| IBIS file stm32l4r5_s5_r7_s7_lqfp144.ibs
[IBIS ver]   4.2
[File name]   stm32l4r5_s5_r7_s7_lqfp144.ibs
[File Rev]   1.0
[Date]   01-6-2017
[Source]   Data Created at STMicroelectronics
[Notes]   File originated from ELDO simulations.
[Disclaimer]  This information is for modeling purpose only and is
   not guaranted.
   The information is subject to change without notice.
[Copyright]   Copyright 2017 STMicroelectronics Inc.
|   Component stm32l4r5_s5_r7_s7_lqfp144
[Component] stm32l4r5_s5_r7_s7_lqfp144
[Manufacturer] STMicroelectronics
[Package]
| variable   typ   min   max
R_pkg   0.0   0.0   0.0
L_pkg   0.0H   0.0H   0.0H
C_pkg   0.0F   0.0F   0.0F
[Pin]  signal_name   model_name   R_pin   L_pin   C_pin
1 PE2 io8prog2m25m50m120m_sudq_ft 187.6E-3 9.4E-9 267.9E-15
2 PE3 io8prog2m25m50m120m_sudq_ft 182.4E-3 9.1E-9 243.8E-15
3 PE4 io8prog2m25m50m120m_sudq_ft 177.6E-3 8.7E-9 221.3E-15
4 PE5 io8prog2m25m50m120m_sudq_ft 173.1E-3 8.4E-9 200.2E-15
5 PE6 io8prog2m25m50m120m_sudq_ft 168.9E-3 8.1E-9 180.5E-15
6 VBAT power 165.0E-3 7.8E-9 162.3E-15
7 PC13 io8prog2m25m50m120m_sudq_ft 161.5E-3 7.6E-9 145.6E-15
8 PC14-OSC32_IN io8prog2m25m50m120m_sudq_ft 158.2E-3 7.4E-9 130.3E-15
9 PC15-OSC32_OUT io8prog2m25m50m120m_sudq_ft 155.2E-3 7.2E-9 116.4E-15
10 PF0 io8prog2m25m50m120m_sudq_i2c_ft 152.6E-3 7.0E-9 104.1E-15
11 PF1 io8prog2m25m50m120m_sudq_i2c_ft 150.3E-3 6.8E-9 93.2E-15
12 PF2 io8prog2m25m50m120m_sudq_ft 148.2E-3 6.7E-9 83.7E-15
13 PF3 io8prog2m25m50m120m_sudq_ft 146.5E-3 6.5E-9 75.7E-15
14 PF4 io8prog2m25m50m120m_sudq_ft 145.1E-3 6.4E-9 69.1E-15
15 PF5 io8prog2m25m50m120m_sudq_ft 144.1E-3 6.4E-9 64.0E-15
16 VSS gnd 143.3E-3 6.3E-9 60.4E-15
17 VDD power 142.8E-3 6.3E-9 58.2E-15
18 PF6 io8prog2m25m50m120m_sudq_ft 142.7E-3 6.3E-9 57.5E-15
19 PF7 io8prog2m25m50m120m_sudq_ft 142.7E-3 6.3E-9 57.5E-15
20 PF8 io8prog2m25m50m120m_sudq_ft 142.8E-3 6.3E-9 58.2E-15
21 PF9 io8prog2m25m50m120m_sudq_ft 143.3E-3 6.3E-9 60.4E-15
22 PF10 io8prog2m25m50m120m_sudq_ft 144.1E-3 6.4E-9 64.0E-15
23 PH0-OSC_IN io8prog2m25m50m120m_sudq_ft 145.1E-3 6.4E-9 69.1E-15
24 PH1-OSC_OUT io8prog2m25m50m120m_sudq_ft 146.5E-3 6.5E-9 75.7E-15
25 NRST ioreset_ft_v33 148.2E-3 6.7E-9 83.7E-15
26 PC0 io8prog2m25m50m120m_sudq_i2c_ft 150.3E-3 6.8E-9 93.2E-15
27 PC1 io8prog2m25m50m120m_sudq_i2c_ft 152.6E-3 7.0E-9 104.1E-15
28 PC2 io8prog2m25m50m120m_sudq_ft 155.2E-3 7.2E-9 116.4E-15
29 PC3 io8prog2m25m50m120m_sudq_ft 158.2E-3 7.4E-9 130.3E-15
30 VSSA gnd 161.5E-3 7.6E-9 145.6E-15
31 VREF- gnd 165.0E-3 7.8E-9 162.3E-15
32 VREF+ power 168.9E-3 8.1E-9 180.5E-15
33 VDDA power 173.1E-3 8.4E-9 200.2E-15
34 PA0 io8prog2m25m50m120m_sudq_ft 177.6E-3 8.7E-9 221.3E-15
35 PA1 io8prog2m25m50m120m_sudq_ft 182.4E-3 9.1E-9 243.8E-15
36 PA2 io8prog2m25m50m120m_sudq_ft 187.6E-3 9.4E-9 267.9E-15
37 PA3 io8prog2m25m50m120m_sudq_ft 187.6E-3 9.4E-9 267.9E-15
38 VSS gnd 182.4E-3 9.1E-9 243.8E-15
39 VDD power 177.6E-3 8.7E-9 221.3E-15
40 PA4 io8prog2m25m50m120m_sudq_ft 173.1E-3 8.4E-9 200.2E-15
41 PA5 io8prog2m25m50m120m_sudq_ft 168.9E-3 8.1E-9 180.5E-15
42 PA6 io8prog2m25m50m120m_sudq_ft 165.0E-3 7.8E-9 162.3E-15
43 PA7 io8prog2m25m50m120m_sudq_i2c_ft 161.5E-3 7.6E-9 145.6E-15
44 PC4 io8prog2m25m50m120m_sudq_ft 158.2E-3 7.4E-9 130.3E-15
45 PC5 io8prog2m25m50m120m_sudq_ft 155.2E-3 7.2E-9 116.4E-15
46 PB0 io8prog2m25m50m120m_sudq_ft 152.6E-3 7.0E-9 104.1E-15
47 PB1 io8prog2m25m50m120m_sudq_ft 150.3E-3 6.8E-9 93.2E-15
48 PB2 io8prog2m25m50m120m_sudq_ft 148.2E-3 6.7E-9 83.7E-15
49 PF11 io8prog2m25m50m120m_sudq_ft 146.5E-3 6.5E-9 75.7E-15
50 PF12 io8prog2m25m50m120m_sudq_ft 145.1E-3 6.4E-9 69.1E-15
51 VSS gnd 144.1E-3 6.4E-9 64.0E-15
52 VDD power 143.3E-3 6.3E-9 60.4E-15
53 PF13 io8prog2m25m50m120m_sudq_ft 142.8E-3 6.3E-9 58.2E-15
54 PF14 io8prog2m25m50m120m_sudq_i2c_ft 142.7E-3 6.3E-9 57.5E-15
55 PF15 io8prog2m25m50m120m_sudq_i2c_ft 142.7E-3 6.3E-9 57.5E-15
56 PG0 io8prog2m25m50m120m_sudq_ft 142.8E-3 6.3E-9 58.2E-15
57 PG1 io8prog2m25m50m120m_sudq_ft 143.3E-3 6.3E-9 60.4E-15
58 PE7 io8prog2m25m50m120m_sudq_ft 144.1E-3 6.4E-9 64.0E-15
59 PE8 io8prog2m25m50m120m_sudq_ft 145.1E-3 6.4E-9 69.1E-15
60 PE9 io8prog2m25m50m120m_sudq_ft 146.5E-3 6.5E-9 75.7E-15
61 VSS gnd 148.2E-3 6.7E-9 83.7E-15
62 VDD power 150.3E-3 6.8E-9 93.2E-15
63 PE10 io8prog2m25m50m120m_sudq_ft 152.6E-3 7.0E-9 104.1E-15
64 PE11 io8prog2m25m50m120m_sudq_ft 155.2E-3 7.2E-9 116.4E-15
65 PE12 io8prog2m25m50m120m_sudq_ft 158.2E-3 7.4E-9 130.3E-15
66 PE13 io8prog2m25m50m120m_sudq_ft 161.5E-3 7.6E-9 145.6E-15
67 PE14 io8prog2m25m50m120m_sudq_ft 165.0E-3 7.8E-9 162.3E-15
68 PE15 io8prog2m25m50m120m_sudq_ft 168.9E-3 8.1E-9 180.5E-15
69 PB10 io8prog2m25m50m120m_sudq_i2c_ft 173.1E-3 8.4E-9 200.2E-15
70 PB11 io8prog2m25m50m120m_sudq_i2c_ft 177.6E-3 8.7E-9 221.3E-15
71 VSS gnd 182.4E-3 9.1E-9 243.8E-15
72 VDD power 187.6E-3 9.4E-9 267.9E-15
73 PB12 io8prog2m25m50m120m_sudq_ft 187.6E-3 9.4E-9 267.9E-15
74 PB13 io8prog2m25m50m120m_sudq_i2c_ft 182.4E-3 9.1E-9 243.8E-15
75 PB14 io8prog2m25m50m120m_sudq_i2c_ft 177.6E-3 8.7E-9 221.3E-15
76 PB15 io8prog2m25m50m120m_sudq_ft 173.1E-3 8.4E-9 200.2E-15
77 PD8 io8prog2m25m50m120m_sudq_ft 168.9E-3 8.1E-9 180.5E-15
78 PD9 io8prog2m25m50m120m_sudq_ft 165.0E-3 7.8E-9 162.3E-15
79 PD10 io8prog2m25m50m120m_sudq_ft 161.5E-3 7.6E-9 145.6E-15
80 PD11 io8prog2m25m50m120m_sudq_ft 158.2E-3 7.4E-9 130.3E-15
81 PD12 io8prog2m25m50m120m_sudq_ft 155.2E-3 7.2E-9 116.4E-15
82 PD13 io8prog2m25m50m120m_sudq_ft 152.6E-3 7.0E-9 104.1E-15
83 VSS gnd 150.3E-3 6.8E-9 93.2E-15
84 VDD power 148.2E-3 6.7E-9 83.7E-15
85 PD14 io8prog2m25m50m120m_sudq_ft 146.5E-3 6.5E-9 75.7E-15
86 PD15 io8prog2m25m50m120m_sudq_ft 145.1E-3 6.4E-9 69.1E-15
87 PG2 io8prog2m25m50m120m_sudq_ft 144.1E-3 6.4E-9 64.0E-15
88 PG3 io8prog2m25m50m120m_sudq_ft 143.3E-3 6.3E-9 60.4E-15
89 PG4 io8prog2m25m50m120m_sudq_ft 142.8E-3 6.3E-9 58.2E-15
90 PG5 io8prog2m25m50m120m_sudq_ft 142.7E-3 6.3E-9 57.5E-15
91 PG6 io8prog2m25m50m120m_sudq_ft 142.7E-3 6.3E-9 57.5E-15
92 PG7 io8prog2m25m50m120m_sudq_i2c_ft 142.8E-3 6.3E-9 58.2E-15
93 PG8 io8prog2m25m50m120m_sudq_i2c_ft 143.3E-3 6.3E-9 60.4E-15
94 VSS gnd 144.1E-3 6.4E-9 64.0E-15
95 VDDIO2 power 145.1E-3 6.4E-9 69.1E-15
96 PC6 io8prog2m25m50m120m_sudq_ft 146.5E-3 6.5E-9 75.7E-15
97 PC7 io8prog2m25m50m120m_sudq_ft 148.2E-3 6.7E-9 83.7E-15
98 PC8 io8prog2m25m50m120m_sudq_ft 150.3E-3 6.8E-9 93.2E-15
99 PC9 io8prog2m25m50m120m_sudq_ft 152.6E-3 7.0E-9 104.1E-15
100 PA8 io8prog2m25m50m120m_sudq_ft 155.2E-3 7.2E-9 116.4E-15
101 PA9 power 158.2E-3 7.4E-9 130.3E-15
102 PA10 io8usb_id_otg20_lcd4_ft_ms 161.5E-3 7.6E-9 145.6E-15
103 PA11 io8usblsfs_otg2 165.0E-3 7.8E-9 162.3E-15
104 PA12 io8usblsfs_otg2 168.9E-3 8.1E-9 180.5E-15
105 PA13 io8prog2m25m50m120m_sudq_ft 173.1E-3 8.4E-9 200.2E-15
106 VDDUSB power 177.6E-3 8.7E-9 221.3E-15
107 VSS gnd 182.4E-3 9.1E-9 243.8E-15
108 VDD power 187.6E-3 9.4E-9 267.9E-15
109 PA14 io8prog2m25m50m120m_sudq_ft 187.6E-3 9.4E-9 267.9E-15
110 PA15 io8prog2m25m50m120m_sudq_ft 182.4E-3 9.1E-9 243.8E-15
111 PC10 io8prog2m25m50m120m_sudq_ft 177.6E-3 8.7E-9 221.3E-15
112 PC11 io8prog2m25m50m120m_sudq_ft 173.1E-3 8.4E-9 200.2E-15
113 PC12 io8prog2m25m50m120m_sudq_ft 168.9E-3 8.1E-9 180.5E-15
114 PD0 io8prog2m25m50m120m_sudq_ft 165.0E-3 7.8E-9 162.3E-15
115 PD1 io8prog2m25m50m120m_sudq_ft 161.5E-3 7.6E-9 145.6E-15
116 PD2 io8prog2m25m50m120m_sudq_ft 158.2E-3 7.4E-9 130.3E-15
117 PD3 io8prog2m25m50m120m_sudq_ft 155.2E-3 7.2E-9 116.4E-15
118 PD4 io8prog2m25m50m120m_sudq_ft 152.6E-3 7.0E-9 104.1E-15
119 PD5 io8prog2m25m50m120m_sudq_ft 150.3E-3 6.8E-9 93.2E-15
120 VSS gnd 148.2E-3 6.7E-9 83.7E-15
121 VDD power 146.5E-3 6.5E-9 75.7E-15
122 PD6 io8prog2m25m50m120m_sudq_ft 145.1E-3 6.4E-9 69.1E-15
123 PD7 io8prog2m25m50m120m_sudq_ft 144.1E-3 6.4E-9 64.0E-15
124 PG9 io8prog2m25m50m120m_sudq_ft 143.3E-3 6.3E-9 60.4E-15
125 PG10 io8prog2m25m50m120m_sudq_ft 142.8E-3 6.3E-9 58.2E-15
126 PG11 io8prog2m25m50m120m_sudq_ft 142.7E-3 6.3E-9 57.5E-15
127 PG12 io8prog2m25m50m120m_sudq_ft 142.7E-3 6.3E-9 57.5E-15
128 PG13 io8prog2m25m50m120m_sudq_i2c_ft 142.8E-3 6.3E-9 58.2E-15
129 PG14 io8prog2m25m50m120m_sudq_i2c_ft 143.3E-3 6.3E-9 60.4E-15
130 VSS gnd 144.1E-3 6.4E-9 64.0E-15
131 VDDIO2 power 145.1E-3 6.4E-9 69.1E-15
132 PG15 io8prog2m25m50m120m_sudq_ft 146.5E-3 6.5E-9 75.7E-15
133 PB3 io8prog2m25m50m120m_sudq_ft 148.2E-3 6.7E-9 83.7E-15
134 PB4 io8prog2m25m50m120m_sudq_i2c_ft 150.3E-3 6.8E-9 93.2E-15
135 PB5 io8prog2m25m50m120m_sudq_ft 152.6E-3 7.0E-9 104.1E-15
136 PB6 io8prog2m25m50m120m_sudq_i2c_ft 155.2E-3 7.2E-9 116.4E-15
137 PB7 io8prog2m25m50m120m_sudq_i2c_ft 158.2E-3 7.4E-9 130.3E-15
138 PH3-BOOT0 io8prog2m25m50m120m_sudq_ft 161.5E-3 7.6E-9 145.6E-15
139 PB8 io8prog2m25m50m120m_sudq_i2c_ft 165.0E-3 7.8E-9 162.3E-15
140 PB9 io8prog2m25m50m120m_sudq_i2c_ft 168.9E-3 8.1E-9 180.5E-15
141 PE0 io8prog2m25m50m120m_sudq_ft 173.1E-3 8.4E-9 200.2E-15
142 PE1 io8prog2m25m50m120m_sudq_ft 177.6E-3 8.7E-9 221.3E-15
143 VSS gnd 182.4E-3 9.1E-9 243.8E-15
144 VDD power 187.6E-3 9.4E-9 267.9E-15
[Diff Pin]   inv_pin   vdiff   tdelay_typ  tdelay_min  tdelay_max
103 104 200mV   NA   NA   NA
[Model Selector] io8prog2m25m50m120m_sudq_ft
io8p00_sudq_ft_pd_lv  "SPEED00, PD=40kOhm - 1P8V"
io8p00_sudq_ft_pu_lv  "SPEED00, PU=40kOhm - 1P8V"
io8p00_sudq_ft_lv  "SPEED00 - 1P8V"
io8p00_sudq_ft_pd  "SPEED00, PD=40kOhm - 3P3V"
io8p00_sudq_ft_pu  "SPEED00, PU=40kOhm - 3P3V"
io8p00_sudq_ft  "SPEED00 - 3P3V"
io8p01_sudq_ft_pd_lv  "SPEED01, PD=40kOhm - 1P8V"
io8p01_sudq_ft_pu_lv  "SPEED01, PU=40kOhm - 1P8V"
io8p01_sudq_ft_lv  "SPEED01 - 1P8V"
io8p01_sudq_ft_pd  "SPEED01, PD=40kOhm - 3P3V"
io8p01_sudq_ft_pu  "SPEED01, PU=40kOhm - 3P3V"
io8p01_sudq_ft  "SPEED01 - 3P3V"
io8p10_sudq_ft_pd_lv  "SPEED10, PD=40kOhm - 1P8V"
io8p10_sudq_ft_pu_lv  "SPEED10, PU=40kOhm - 1P8V"
io8p10_sudq_ft_lv  "SPEED10 - 1P8V"
io8p10_sudq_ft_pd  "SPEED10, PD=40kOhm - 3P3V"
io8p10_sudq_ft_pu  "SPEED10, PU=40kOhm - 3P3V"
io8p10_sudq_ft  "SPEED10 - 3P3V"
io8p11_sudq_ft_pd_lv  "SPEED11, PD=40kOhm - 1P8V"
io8p11_sudq_ft_pu_lv  "SPEED11, PU=40kOhm - 1P8V"
io8p11_sudq_ft_lv  "SPEED11 - 1P8V"
io8p11_sudq_ft_pd  "SPEED11, PD=40kOhm - 3P3V"
io8p11_sudq_ft_pu  "SPEED11, PU=40kOhm - 3P3V"
io8p11_sudq_ft  "SPEED11 - 3P3V"
[Model Selector] io8prog2m25m50m120m_sudq_i2c_ft
io8prog_1v8_i2c_pd  "5V Tol GPIO 1.8V range i2c functionality with pull down"
io8prog_1v8_i2c_pu  "5V Tol GPIO 1.8V range i2c functionality with pull up"
io8prog_1v8_i2c  "5V Tol GPIO 1.8V range i2c functionality"
io8prog_3v3_i2c_pd  "5V Tol GPIO 3.3V range i2c functionality with pull down"
io8prog_3v3_i2c_pu  "5V Tol GPIO 3.3V range i2c functionality with pull up"
io8prog_3v3_i2c  "5V Tol GPIO 3.3V range i2c functionality"
io8prog_1v8_pd_00  "5V Tol GPIO 1.8V range with pd speed 00"
io8prog_1v8_pu_00  "5V Tol GPIO 1.8V range with pu speed 00"
io8prog_1v8_00  "5V Tol GPIO 1.8V range speed 00"
io8prog_3v3_pd_00  "5V Tol GPIO 3.3V range with pd speed 00"
io8prog_3v3_pu_00  "5V Tol GPIO 3.3V range with pu speed 00"
io8prog_3v3_00  "5V Tol GPIO 3.3V range speed 00"
io8prog_1v8_pd_01  "5V Tol GPIO 1.8V range with pd speed 01"
io8prog_1v8_pu_01  "5V Tol GPIO 1.8V range with pu speed 01"
io8prog_1v8_01  "5V Tol GPIO 1.8V range speed 01"
io8prog_3v3_pd_01  "5V Tol GPIO 3.3V range with pd speed 01"
io8prog_3v3_pu_01  "5V Tol GPIO 3.3V range with pu speed 01"
io8prog_3v3_01  "5V Tol GPIO 3.3V range speed 01"
io8prog_1v8_pd_10  "5V Tol GPIO 1.8V range with pd speed 10"
io8prog_1v8_pu_10  "5V Tol GPIO 1.8V range with pu speed 10"
io8prog_1v8_10  "5V Tol GPIO 1.8V range speed 10"
io8prog_3v3_pd_10  "5V Tol GPIO 3.3V range with pd speed 10"
io8prog_3v3_pu_10  "5V Tol GPIO 3.3V range with pu speed 10"
io8prog_3v3_10  "5V Tol GPIO 3.3V range speed 10"
io8prog_1v8_pd_11  "5V Tol GPIO 1.8V range with pd speed 11"
io8prog_1v8_pu_11  "5V Tol GPIO 1.8V range with pu speed 11"
io8prog_1v8_11  "5V Tol GPIO 1.8V range speed 11"
io8prog_3v3_pd_11  "5V Tol GPIO 3.3V range with pd speed 11"
io8prog_3v3_pu_11  "5V Tol GPIO 3.3V range with pu speed 11"
io8prog_3v3_11  "5V Tol GPIO 3.3V range speed 11"
[Model Selector] io8usb_id_otg20_lcd4_ft_ms
io8usbid_1v8_id_pu  "ID 1V8 range with pull up"
io8usbid_3v3_id_pu  "ID 3V3 range with pull up"
io8usbid_1v8_id  "ID 1V8 range"
io8usbid_3v3_id  "ID 3V3 range"
io8usbid_1v8_pd_00  "GPIO 1.8V range with pd speed 00"
io8usbid_1v8_pu_00  "GPIO 1.8V range with pu speed 00"
io8usbid_1v8_00  "GPIO 1.8V range speed 00"
io8usbid_3v3_pd_00  "GPIO 3.3V range with pd speed 00"
io8usbid_3v3_pu_00  "GPIO 3.3V range with pu speed 00"
io8usbid_3v3_00  "GPIO 3.3V range speed 00"
io8usbid_1v8_pd_01  "GPIO 1.8V range with pd speed 01"
io8usbid_1v8_pu_01  "GPIO 1.8V range with pu speed 01"
io8usbid_1v8_01  "GPIO 1.8V range speed 01"
io8usbid_3v3_pd_01  "GPIO 3.3V range with pd speed 01"
io8usbid_3v3_pu_01  "GPIO 3.3V range with pu speed 01"
io8usbid_3v3_01  "GPIO 3.3V range speed 01"
io8usbid_1v8_pd_10  "GPIO 1.8V range with pd speed 10"
io8usbid_1v8_pu_10  "GPIO 1.8V range with pu speed 10"
io8usbid_1v8_10  "GPIO 1.8V range speed 10"
io8usbid_3v3_pd_10  "GPIO 3.3V range with pd speed 10"
io8usbid_3v3_pu_10  "GPIO 3.3V range with pu speed 10"
io8usbid_3v3_10  "GPIO 3.3V range speed 10"
io8usbid_1v8_pd_11  "GPIO 1.8V range with pd speed 11"
io8usbid_1v8_pu_11  "GPIO 1.8V range with pu speed 11"
io8usbid_1v8_11  "GPIO 1.8V range speed 11"
io8usbid_3v3_pd_11  "GPIO 3.3V range with pd speed 11"
io8usbid_3v3_pu_11  "GPIO 3.3V range with pu speed 11"
io8usbid_3v3_11  "GPIO 3.3V range speed 11"
[Model Selector] io8usblsfs_otg2
usb_ls_pd  "USB Low Speed mode - Pull Down"
usb_ls_pu2  "USB Low Speed mode - Pull up 2"
usb_ls_pu  "USB Low Speed mode - Pull up"
usb_fs  "USB Low Speed mode"
usb_fs_pd  "USB Full Speed mode - Pull Down"
usb_fs_pu2  "USB Full Speed mode - Pull up 2"
usb_fs_pu  "USB Full Speed mode - Pull up"
[Model Selector] ioreset_ft_v33
ioreset_1v2_pu  "RESET 1.2V range with PU"
ioreset_1v2  "RESET 1.2V range"
ioreset_1v8_pu  "RESET 1.8V range with PU"
ioreset_1v8  "RESET 1.8V range"
ioreset_3v3_pu  "RESET 3.3V range with PU"
ioreset_3v3  "RESET 3.3V range"
| Models and submodels in the file (95): io8p00_sudq_ft_pd_lv (I/O), io8p00_sudq_ft_pu_lv (I/O), io8p00_sudq_ft_lv (I/O), io8p00_sudq_ft_pd (I/O), io8p00_sudq_ft_pu (I/O), io8p00_sudq_ft (I/O), io8p01_sudq_ft_pd_lv (I/O), io8p01_sudq_ft_pu_lv (I/O), io8p01_sudq_ft_lv (I/O), io8p01_sudq_ft_pd (I/O), io8p01_sudq_ft_pu (I/O), io8p01_sudq_ft (I/O), io8p10_sudq_ft_pd_lv (I/O), io8p10_sudq_ft_pu_lv (I/O), io8p10_sudq_ft_lv (I/O), io8p10_sudq_ft_pd (I/O), io8p10_sudq_ft_pu (I/O), io8p10_sudq_ft (I/O), io8p11_sudq_ft_pd_lv (I/O), io8p11_sudq_ft_pu_lv (I/O), io8p11_sudq_ft_lv (I/O), io8p11_sudq_ft_pd (I/O), io8p11_sudq_ft_pu (I/O), io8p11_sudq_ft (I/O), io8prog_1v8_i2c_pd (I/O), io8prog_1v8_i2c_pu (I/O), io8prog_1v8_i2c (I/O), io8prog_3v3_i2c_pd (I/O), io8prog_3v3_i2c_pu (I/O), io8prog_3v3_i2c (I/O), io8prog_1v8_pd_00 (I/O), io8prog_1v8_pu_00 (I/O), io8prog_1v8_00 (I/O), io8prog_3v3_pd_00 (I/O), io8prog_3v3_pu_00 (I/O), io8prog_3v3_00 (I/O), io8prog_1v8_pd_01 (I/O), io8prog_1v8_pu_01 (I/O), io8prog_1v8_01 (I/O), io8prog_3v3_pd_01 (I/O), io8prog_3v3_pu_01 (I/O), io8prog_3v3_01 (I/O), io8prog_1v8_pd_10 (I/O), io8prog_1v8_pu_10 (I/O), io8prog_1v8_10 (I/O), io8prog_3v3_pd_10 (I/O), io8prog_3v3_pu_10 (I/O), io8prog_3v3_10 (I/O), io8prog_1v8_pd_11 (I/O), io8prog_1v8_pu_11 (I/O), io8prog_1v8_11 (I/O), io8prog_3v3_pd_11 (I/O), io8prog_3v3_pu_11 (I/O), io8prog_3v3_11 (I/O), io8usbid_1v8_id_pu (Input), io8usbid_3v3_id_pu (Input), io8usbid_1v8_id (Input), io8usbid_3v3_id (Input), io8usbid_1v8_pd_00 (I/O), io8usbid_1v8_pu_00 (I/O), io8usbid_1v8_00 (I/O), io8usbid_3v3_pd_00 (I/O), io8usbid_3v3_pu_00 (I/O), io8usbid_3v3_00 (I/O), io8usbid_1v8_pd_01 (I/O), io8usbid_1v8_pu_01 (I/O), io8usbid_1v8_01 (I/O), io8usbid_3v3_pd_01 (I/O), io8usbid_3v3_pu_01 (I/O), io8usbid_3v3_01 (I/O), io8usbid_1v8_pd_10 (I/O), io8usbid_1v8_pu_10 (I/O), io8usbid_1v8_10 (I/O), io8usbid_3v3_pd_10 (I/O), io8usbid_3v3_pu_10 (I/O), io8usbid_3v3_10 (I/O), io8usbid_1v8_pd_11 (I/O), io8usbid_1v8_pu_11 (I/O), io8usbid_1v8_11 (I/O), io8usbid_3v3_pd_11 (I/O)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
